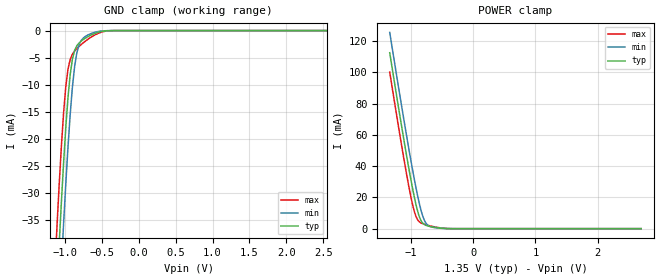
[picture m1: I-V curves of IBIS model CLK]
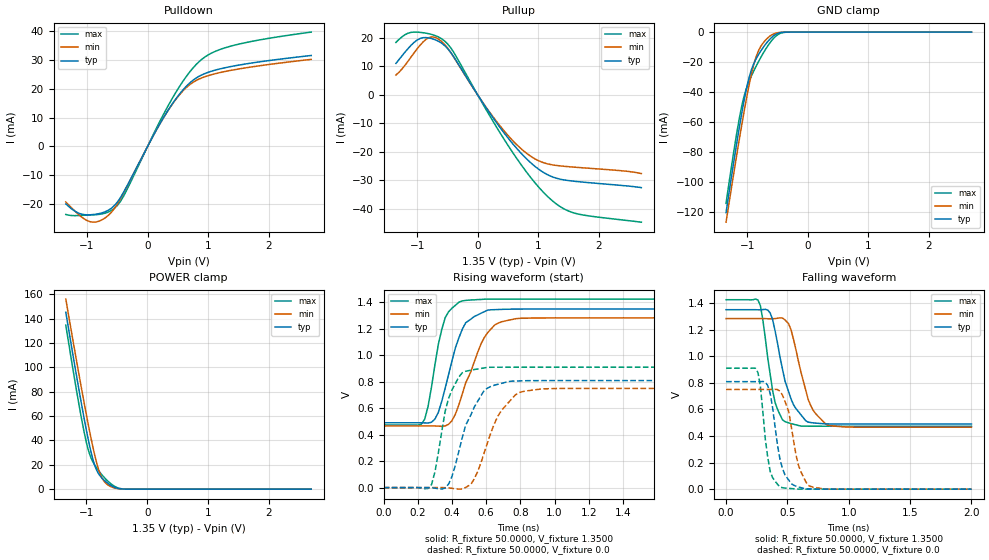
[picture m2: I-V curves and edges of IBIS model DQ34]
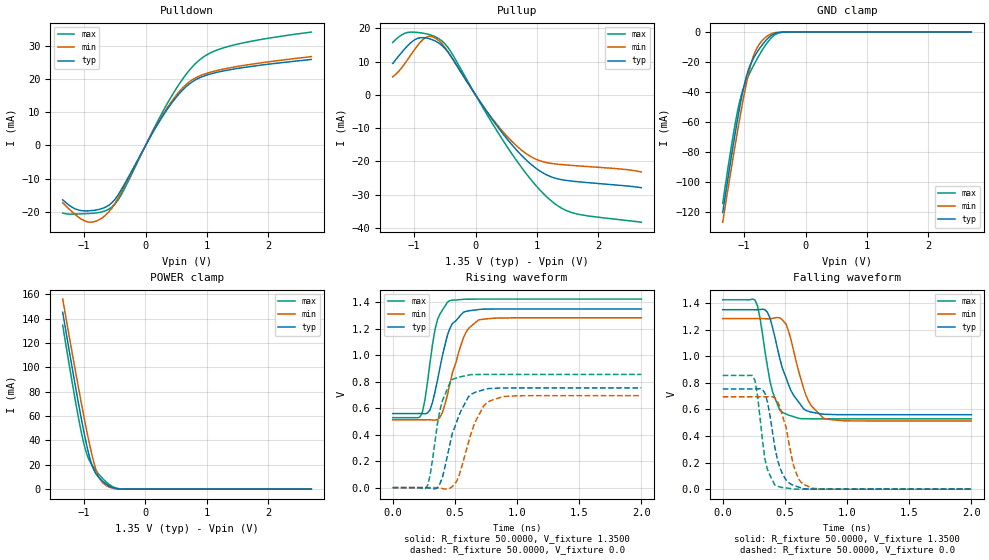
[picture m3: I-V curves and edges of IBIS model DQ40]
|   IBIS file usslh2g16ec.ibs
[IBIS ver] 3.2
[File name] usslh2g16ec.ibs
[File Rev] 1.06
[Date] Dec. 08th, 2020
[Source] File generated by UniIC.
[Notes]  Rev 1.0: 03/21/2019
   - New model generated.
   Rev 1.01: 06/12/2019
   - Adjust DQ34/DQ40 model rising waveform and
   falling waveform.
   Rev 1.02: 10/03/2019
   - 1. Modify CLK and INPUT model GND Clamp and POWER Clamp.
   - 2. Moidfy DQ34 and DQ40 model.
   Rev 1.03: 12/06/2019
   - Modified all ODT model content. Change to use v1.0 value.
   Rev 1.04: 12/06/2019
   - Update RLC information.
   Rev 1.05: 12/23/2019
   - Modified content of all ODT models.
   Rev 1.06: 12/08/2020
   - update 95c data.
[Disclaimer]  THESE IBIS MODELS ARE PROVIDED "AS IS" WITH NO WARRANTY
   AND UniIC IS NOT RESPONSIBLE FOR ANY PROBLEMS THIS MODEL
   MAY CAUSE TO THE CUSTOMERS. THESE MODELS ARE SUBJECT TO CHANGE
   WITHOUT ANY NOTICE.
[Copyright] Copyright 2020. UniIC All rights reserved.
|   Component: SCB13H2G160EF
|   2G DDR3L SDRAM X16
|   VDD/VDDQ : 1.35V
[Component] SCB13H2G160EF
[Manufacturer]  UniIC.
[Package]
|   typ   min   max
R_pkg   0.624   0.464   0.798
L_pkg   1.862nH   1.145nH   3.060nH
C_pkg   0.529pF   0.376pF   0.813pF
[Pin]   signal_name   model_name   R_pin   L_pin   C_pin
A1   VDDQ   POWER
A2   DQU5   DQ   0.782   2.212nH   0.593pF
A3   DQU7   DQ   0.720   1.890nH   0.554pF
A7   DQU4   DQ   0.536   1.899nH   0.568pF
A8   VDDQ   POWER
A9   VSS   GND
B1   VSS   GND
B2   VDD   POWER
B3   VSS   GND
B7   DQSUB   DQ   0.674   1.734nH   0.587pF
B8   DQU6   DQ   0.791   2.263nH   0.576pF
B9   VSS   GND
C1   VDDQ   POWER
C2   DQU3   DQ   0.669   1.891nH   0.538pF
C3   DQU1   DQ   0.577   1.375nH   0.563pF
C7   DQSU   DQ   0.678   1.680nH   0.578pF
C8   DQU2   DQ   0.759   2.136nH   0.557pF
C9   VDDQ   POWER
D1   VSS   GND
D2   VDDQ   POWER
D3   DMU   DQ   0.570   1.24nH   0.562pF
D7   DQU0   DQ   0.511   1.214nH   0.532pF
D8   VSS   GND
D9   VDD   POWER
E1   VSS   GND
E2   VSS   GND
E3   DQL0   DQ   0.527   1.246nH   0.558pF
E7   DML   DQ   0.528   1.181nH   0.559pF
E8   VSS   GND
E9   VDDQ   POWER
F1   VDDQ   POWER
F2   DQL2   DQ   0.649   1.448nH   0.569pF
F3   DQSL   DQ   0.600   1.602nH   0.552pF
F7   DQL1   DQ   0.503   1.145nH   0.544pF
F8   DQL3   DQ   0.610   1.407nH   0.554pF
F9   VSS   GND
G1   VSS   GND
G2   DQL6   DQ   0.589   1.311nH   0.543pF
G3   DQSLB   DQ   0.595   1.638nH   0.544pF
G7   VDD   POWER
G8   VSS   GND
G9   VSS   GND
H1   VREFQ   POWER
H2   VDD   POWER
H3   DQL4   DQ   0.550   1.26nH   0.565pF
H7   DQL7   DQ   0.587   1.352nH   0.567pF
H8   DQL5   DQ   0.731   1.671nH   0.576pF
H9   VDDQ   POWER
J2   VSS   GND
J3   RASB   INPUT   0.464   1.391nH   0.444pF
J7   CK   CLK   0.472   1.167nH   0.376pF
J8   VSS   GND
K1   ODT   INPUT   0.628   2.345nH   0.451pF
K2   VDD   POWER
K3   CASB   INPUT   0.476   1.52nH   0.452pF
K7   CKB   CLK   0.467   1.314nH   0.389pF
K8   VDD   POWER
K9   CKE   INPUT   0.685   2.271nH   0.502pF
L2   CSB   INPUT   0.576   2.026nH   0.444pF
L3   WEB   INPUT   0.495   1.669nH   0.437pF
L7   A10   INPUT   0.491   1.335nH   0.448pF
L8   ZQ   INPUT   0.652   1.676nH   0.497pF
M1   VSS   GND
M2   BA0   INPUT   0.601   2.209nH   0.446pF
M3   BA2   INPUT   0.565   1.827nH   0.450pF
M9   VSS   GND
N1   VDD   POWER
N2   A3   INPUT   0.669   2.297nH   0.501pF
N3   A0   INPUT   0.546   1.663nH   0.460pF
N7   A12   INPUT   0.545   1.919nH   0.480pF
N8   BA1   INPUT   0.671   2.186nH   0.501pF
N9   VDD   POWER
P1   VSS   GND
P2   A5   INPUT   0.701   2.412nH   0.530pF
P3   A2   INPUT   0.614   2.102nH   0.542pF
P7   A1   INPUT   0.582   2.095nH   0.521pF
P8   A4   INPUT   0.686   2.439nH   0.542pF
P9   VSS   GND
R1   VSS   GND
R2   A7   INPUT   0.763   2.744nH   0.587pF
R3   A9   INPUT   0.673   2.375nH   0.534pF
R7   A11   INPUT   0.633   2.347nH   0.507pF
R8   A6   INPUT   0.761   2.758nH   0.599pF
R9   VDD   POWER
T1   VSS   GND
T2   RESETB   INPUT   0.798   2.031nH   0.813pF
T3   A13   INPUT   0.752   2.571nH   0.549pF
T7   A14   INPUT   0.717   2.562nH   0.523pF
T8   A8   INPUT   0.798   3.060nH   0.580pF
T9   VSS   GND
|**********************DIFF PIN*********************************************
[Diff_pin]   inv_pin   vdiff   tdelay_typ   tdelay_min   tdelay_max
   J7   K7   0V   0ns   NA   NA
   F3   G3   0V   0ns   NA   NA
   C7   B7   0V   0ns   NA   NA
|   Model Selector
[Model Selector]  DQ
DQ34   34ohm data I/O without ODT
DQ40   40ohm data I/O without ODT
ODT20   Data input with 20ohm ODT
ODT30   Data input with 30ohm ODT
ODT40   Data input with 40ohm ODT
ODT60   Data input with 60ohm ODT
ODT120   Data input with 120ohm ODT
| Models and submodels in the file (14): CLK (Input), INPUT (Input), DQ34 (I/O), DQ40 (I/O), ODT20 (Input), ODT30 (Input), ODT40 (Input), ODT60 (Input), ODT120 (Input), 20ohm_ODT (Dynamic_clamp), 30ohm_ODT (Dynamic_clamp), 40ohm_ODT (Dynamic_clamp), 60ohm_ODT (Dynamic_clamp), 120ohm_ODT (Dynamic_clamp)
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|   Model CLK
[Model]  CLK
Model_type   Input
Polarity   Non-Inverting
Vinl =   0.5750V
Vinh =   0.7750V
| variable   typ   min   max
C_comp   0.4980pF   0.4480pF   0.5480pF
| variable   typ   min   max
[Temperature Range]   45.000   95.000   0.000
| variable   typ   min   max
[Voltage Range]   1.35V   1.283V   1.4250V
| variable   typ   min   max
[POWER Clamp Reference] 1.35V   1.283V   1.4250V
| variable   typ   min   max
[GND Clamp Reference]   0.000V   0.000V   0.000V
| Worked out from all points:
|   GND clamp passes 1 mA (typ) near -0.67 V on its own axis
|   POWER clamp passes 1 mA (typ) near -0.64 V on its own axis
[GND_clamp]
|Voltage   I(typ)   I(min)   I(max)
-1.35V    -119.8mA   -132.6mA   -107.8mA
-1.11V    -47.85mA   -60.25mA   -36.41mA
-1.08V    -39.66mA   -51.82mA   -28.64mA
-1.05V    -31.85mA   -43.65mA   -21.5mA
-1.02V    -24.55mA   -35.8mA    -15.28mA
-990mV    -17.97mA   -28.39mA   -10.4mA
-930mV    -8.108mA   -15.48mA   -5.33mA
-870mV    -3.674mA   -6.627mA   -3.777mA
-810mV    -2.286mA   -2.636mA   -2.929mA
-720mV    -1.363mA   -1.035mA   -1.906mA
-390mV    -14.42uA   -7.911uA   -27.31uA
2.7V      0A         0A         0A
[POWER_clamp]
|Voltage   I(typ)   I(min)   I(max)
-1.34V    112.5mA    125.5mA    100.1mA
-1.2V     77.82mA    90.79mA    65.48mA
-1.1V     53.88mA    66.67mA    41.81mA
-1.02V    35.69mA    48.08mA    24.36mA
-960mV    23.14mA    34.83mA    13.32mA
-900mV    12.44mA    22.6mA     6.231mA
-840mV    5.342mA    12.19mA    3.716mA
-780mV    2.549mA    5.064mA    2.758mA
-720mV    1.647mA    1.95mA     2.065mA
-600mV    737.4uA    566.8uA    984.4uA
-360mV    19.27uA    12.95uA    28.6uA
2.7V      0A         0A         0A
|   Model DQ34
[Model]  DQ34
Model_type I/O
Polarity   Non-Inverting
Enable   Active-High
Vinl =   0.5750V
Vinh =   0.7750V
Vmeas =  0.6750V
Cref =   0.0F
Rref =   25.0000
Vref =   0.6750V
| variable   typ   min   max
C_comp   1.0500pF   1.0000pF   1.1000pF
| variable   typ   min   max
[Temperature Range]   45.000   95.000   0.000
| variable   typ   min   max
[Voltage Range]   1.35V   1.283V   1.4250V
| variable   typ   min   max
[Pullup Reference]   1.35V   1.283V   1.4250V
| variable   typ   min   max
[Pulldown Reference]   0.000V   0.000V   0.000V
| variable   typ   min   max
[POWER Clamp Reference] 1.35V   1.283V   1.4250V
| variable   typ   min   max
[GND Clamp Reference]   0.000V   0.000V   0.000V
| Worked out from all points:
|   slope of the pulldown table from 0 to 0.203 V, typ, clamps not added: 25.8 ohm
|   slope of the pullup table from 0 to 0.203 V, typ, clamps not added: 31.3 ohm
|   GND clamp passes 1 mA (typ) near -0.50 V on its own axis
|   POWER clamp passes 1 mA (typ) near -0.51 V on its own axis
|   rising waveform, R_fixture 50.0000, V_fixture 1.3500: 20-80 % time 112ps typ, 142ps min, 82.2ps max; typ from 0.49 V to 1.35 V
|   rising waveform, R_fixture 50.0000, V_fixture 0.0: 20-80 % time 130ps typ, 142ps min, 87.7ps max; typ from 0 V to 0.809 V
|   falling waveform, R_fixture 50.0000, V_fixture 1.3500: 20-80 % time 135ps typ, 138ps min, 91.5ps max; typ from 1.35 V to 0.49 V
|   falling waveform, R_fixture 50.0000, V_fixture 0.0: 20-80 % time 84.9ps typ, 97.5ps min, 66ps max; typ from 0.809 V to 0 V
[Pulldown]
|Voltage   I(typ)   I(min)   I(max)
-1.35V    -19.97mA   -19.29mA   -23.65mA
-1.15V    -23.09mA   -23.47mA   -24.03mA
-950mV    -23.77mA   -26.17mA   -23.85mA
-650mV    -22.21mA   -24.01mA   -22.83mA
-500mV    -19.4mA    -20.05mA   -20.54mA
-400mV    -16.07mA   -16.29mA   -17.41mA
100mV     3.983mA    3.979mA    4.397mA
400mV     14.55mA    14.43mA    16.42mA
650mV     21.14mA    20.67mA    24.63mA
900mV     24.9mA     23.86mA    30.36mA
1.45V     28.05mA    26.72mA    35.27mA
2.7V      31.59mA    30.25mA    39.73mA
[Pullup]
|Voltage   I(typ)   I(min)   I(max)
-1.35V    11.07mA    6.98mA     18.44mA
-1.15V    16.28mA    11.86mA    21.68mA
-1V       19.27mA    16.18mA    22.06mA
-850mV    20.14mA    19.59mA    21.68mA
-700mV    19.35mA    20.18mA    20.83mA
-400mV    13.51mA    13.42mA    15.11mA
150mV     -4.843mA   -4.665mA   -5.558mA
550mV     -16.41mA   -15.39mA   -19.33mA
900mV     -24.27mA   -21.87mA   -29.66mA
1.2V      -28.46mA   -24.4mA    -36.56mA
1.6V      -30.3mA    -25.34mA   -41.48mA
2.7V      -32.52mA   -27.58mA   -44.65mA
[GND_clamp]
|Voltage   I(typ)   I(min)   I(max)
-1.35V    -120.2mA   -126.6mA   -114.1mA
-1.23V    -88.34mA   -95.9mA    -81.52mA
-1.14V    -65.66mA   -73.61mA   -59.5mA
-1.05V    -45.07mA   -52.44mA   -42.33mA
-990mV    -33.57mA   -39.39mA   -34.75mA
-930mV    -24.92mA   -27.79mA   -29.03mA
-840mV    -16.77mA   -14.89mA   -21.65mA
-750mV    -10.97mA   -7.891mA   -14.99mA
-630mV    -4.83mA    -2.8mA     -7.385mA
-510mV    -1.116mA   -502.7uA   -2.115mA
-360mV    -46.72uA   -22.21uA   -95.74uA
2.7V      0A         0A         0A
[POWER_clamp]
|Voltage   I(typ)   I(min)   I(max)
-1.34V    145.4mA    156.2mA    134.8mA
-1.12V    80.7mA     93.36mA    68.62mA
-1.04V    58.61mA    71.47mA    47.35mA
-980mV    43.17mA    55.66mA    34.17mA
-940mV    33.8mA     45.58mA    27.64mA
-880mV    22.09mA    31.49mA    21.14mA
-800mV    12.67mA    16.11mA    15.22mA
-740mV    8.89mA     8.743mA    11.48mA
-660mV    5.266mA    3.989mA    7.183mA
-520mV    1.208mA    721.2uA    1.904mA
-360mV    46.31uA    30.1uA     72.07uA
2.7V      0A         0A         0A
[Ramp]
| variable   typ   min   max
dV/dt_r  0.4853/0.1200n   0.4499/0.1421n   0.5459/88.0013p
dV/dt_f  0.5160/0.1249n   0.4903/0.1383n   0.5710/91.2670p
R_load = 50.0000
[Rising Waveform]
R_fixture= 50.0000
V_fixture= 1.3500
V_fixture_min= 1.2830
V_fixture_max= 1.4250
L_fixture= 0.0H
C_fixture= 0.0F
|time   V(typ)   V(min)   V(max)
0s        490mV      465.8mV    473.3mV
240ps     489.3mV    465.8mV    516.5mV
260ps     488.1mV    465.8mV    613.9mV
300ps     517.4mV    465.9mV    927.6mV
360ps     751.1mV    466.1mV    1.284V
400ps     958.8mV    505.9mV    1.356V
460ps     1.196V     706.9mV    1.411V
590ps     1.33V      1.136V     1.424V
690ps     1.347V     1.253V     1.425V
2ns       1.35V      1.283V     1.425V
[Rising Waveform]
R_fixture= 50.0000
V_fixture= 0.0
V_fixture_min= 0.0
V_fixture_max= 0.0
L_fixture= 0.0H
C_fixture= 0.0F
|time   V(typ)   V(min)   V(max)
0s        0V         0V         0V
280ps     -938.2uV   -50.3uV    22.28mV
380ps     26.61mV    -2.235mV   674.6mV
440ps     273.8mV    -11.77mV   836mV
480ps     471.5mV    1.462mV    879.3mV
530ps     607.6mV    65.88mV    892.1mV
590ps     737mV      269.6mV    905mV
670ps     781.4mV    542.8mV    909.7mV
790ps     806.3mV    717.3mV    909.9mV
2ns       808.8mV    749.8mV    909.9mV
[Falling Waveform]
R_fixture= 50.0000
V_fixture= 1.3500
V_fixture_min= 1.2830
V_fixture_max= 1.4250
L_fixture= 0.0H
C_fixture= 0.0F
|time   V(typ)   V(min)   V(max)
0s        1.35V      1.283V     1.425V
260ps     1.349V     1.283V     1.423V
300ps     1.351V     1.283V     1.272V
360ps     1.325V     1.282V     862.1mV
400ps     1.189V     1.283V     650.3mV
480ps     815.1mV    1.274V     508.2mV
530ps     677.3mV    1.198V     492.8mV
670ps     503.9mV    672.9mV    473.6mV
830ps     490.9mV    481mV      473.3mV
2ns       490mV      465.8mV    473.3mV
[Falling Waveform]
R_fixture= 50.0000
V_fixture= 0.0
V_fixture_min= 0.0
V_fixture_max= 0.0
L_fixture= 0.0H
C_fixture= 0.0F
|time   V(typ)   V(min)   V(max)
0s        808.8mV    749.8mV    909.9mV
260ps     808.5mV    749.8mV    876.9mV
280ps     808.7mV    749.9mV    772.8mV
320ps     805.7mV    749.8mV    376.4mV
360ps     718.4mV    749.6mV    132.1mV
440ps     222mV      736.8mV    15.22mV
510ps     69.56mV    586.8mV    5.903mV
590ps     16.7mV     179.9mV    358.3uV
670ps     1.797mV    27.86mV    -70.56uV
2ns       1.662uV    -1.338uV   1.858uV
|   Model DQ40
[Model]  DQ40
Model_type I/O
Polarity   Non-Inverting
Enable   Active-High
Vinl =   0.5750V
Vinh =   0.7750V
Vmeas =  0.6750V
Cref =   0.0F
Rref =   25.0000
Vref =   0.6750V
| variable   typ   min   max
C_comp   1.0500pF   1.0000pF   1.1000pF
| variable   typ   min   max
[Temperature Range]   45.000   95.000   0.000
| variable   typ   min   max
[Voltage Range]   1.35V   1.283V   1.4250V
| variable   typ   min   max
[Pullup Reference]   1.35V   1.283V   1.4250V
| variable   typ   min   max
[Pulldown Reference]   0.000V   0.000V   0.000V
| variable   typ   min   max
[POWER Clamp Reference] 1.35V   1.283V   1.4250V
| variable   typ   min   max
[GND Clamp Reference]   0.000V   0.000V   0.000V
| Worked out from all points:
|   slope of the pulldown table from 0 to 0.203 V, typ, clamps not added: 31 ohm
|   slope of the pullup table from 0 to 0.203 V, typ, clamps not added: 36.5 ohm
|   GND clamp passes 1 mA (typ) near -0.50 V on its own axis
|   POWER clamp passes 1 mA (typ) near -0.51 V on its own axis
|   rising waveform, R_fixture 50.0000, V_fixture 1.3500: 20-80 % time 117ps typ, 137ps min, 87.4ps max; typ from 0.56 V to 1.35 V
|   rising waveform, R_fixture 50.0000, V_fixture 0.0: 20-80 % time 143ps typ, 148ps min, 98.7ps max; typ from 0 V to 0.754 V
|   falling waveform, R_fixture 50.0000, V_fixture 1.3500: 20-80 % time 156ps typ, 141ps min, 104ps max; typ from 1.35 V to 0.56 V
|   falling waveform, R_fixture 50.0000, V_fixture 0.0: 20-80 % time 94.4ps typ, 106ps min, 71.5ps max; typ from 0.754 V to 0 V
[Pulldown]
|Voltage   I(typ)   I(min)   I(max)
-1.35V    -16.31mA   -17.17mA   -20.27mA
-1.15V    -19.01mA   -20.69mA   -20.6mA
-950mV    -19.64mA   -22.91mA   -20.44mA
-650mV    -18.49mA   -20.9mA    -19.57mA
-500mV    -16.2mA    -17.43mA   -17.61mA
-400mV    -13.43mA   -14.16mA   -14.92mA
100mV     3.324mA    3.459mA    3.769mA
400mV     12.09mA    12.6mA     14.08mA
650mV     17.49mA    18.14mA    21.11mA
900mV     20.49mA    21.04mA    26.02mA
1.45V     22.99mA    23.58mA    30.23mA
2.7V      25.82mA    26.68mA    34.05mA
[Pullup]
|Voltage   I(typ)   I(min)   I(max)
-1.35V    9.49mA     5.47mA     15.8mA
-1.15V    13.95mA    9.5mA      18.59mA
-1V       16.52mA    13.51mA    18.91mA
-850mV    17.26mA    16.81mA    18.58mA
-700mV    16.59mA    17.5mA     17.86mA
-400mV    11.58mA    11.64mA    12.95mA
150mV     -4.151mA   -4.025mA   -4.764mA
550mV     -14.06mA   -13.18mA   -16.57mA
900mV     -20.81mA   -18.54mA   -25.42mA
1.2V      -24.4mA    -20.49mA   -31.34mA
1.65V     -26.07mA   -21.3mA    -35.79mA
2.7V      -27.88mA   -23.18mA   -38.27mA
[GND_clamp]
|Voltage   I(typ)   I(min)   I(max)
-1.35V    -120.2mA   -126.6mA   -114.1mA
-1.23V    -88.34mA   -95.9mA    -81.52mA
-1.14V    -65.66mA   -73.61mA   -59.5mA
-1.05V    -45.07mA   -52.44mA   -42.33mA
-990mV    -33.57mA   -39.39mA   -34.75mA
-930mV    -24.92mA   -27.79mA   -29.03mA
-840mV    -16.77mA   -14.89mA   -21.65mA
-750mV    -10.97mA   -7.891mA   -14.99mA
-630mV    -4.83mA    -2.8mA     -7.385mA
-510mV    -1.116mA   -502.7uA   -2.115mA
-360mV    -46.72uA   -22.21uA   -95.74uA
2.7V      0A         0A         0A
[POWER_clamp]
|Voltage   I(typ)   I(min)   I(max)
-1.34V    145.4mA    156.2mA    134.8mA
-1.12V    80.7mA     93.36mA    68.62mA
-1.04V    58.61mA    71.47mA    47.35mA
-980mV    43.17mA    55.66mA    34.17mA
-940mV    33.8mA     45.58mA    27.64mA
-880mV    22.09mA    31.49mA    21.14mA
-800mV    12.67mA    16.11mA    15.22mA
-740mV    8.89mA     8.743mA    11.48mA
-660mV    5.266mA    3.989mA    7.183mA
-520mV    1.208mA    721.2uA    1.904mA
-360mV    46.31uA    30.1uA     72.07uA
2.7V      0A         0A         0A
[Ramp]
| variable   typ   min   max
dV/dt_r  0.4523/0.1331n   0.4170/0.1476n   0.5132/98.6582p
dV/dt_f  0.4740/0.1462n   0.4620/0.1406n   0.5376/0.1040n
R_load = 50.0000
[Rising Waveform]
R_fixture= 50.0000
V_fixture= 1.3500
V_fixture_min= 1.2830
V_fixture_max= 1.4250
L_fixture= 0.0H
C_fixture= 0.0F
|time   V(typ)   V(min)   V(max)
0s        560mV      513mV      529mV
220ps     560.2mV    513mV      535mV
260ps     557.7mV    513mV      666.2mV
300ps     588.3mV    513mV      945.1mV
360ps     811.2mV    513.9mV    1.269V
400ps     998.2mV    568.3mV    1.342V
460ps     1.203V     782.9mV    1.414V
570ps     1.326V     1.135V     1.423V
690ps     1.346V     1.267V     1.425V
2ns       1.35V      1.283V     1.425V
[Rising Waveform]
R_fixture= 50.0000
V_fixture= 0.0
V_fixture_min= 0.0
V_fixture_max= 0.0
L_fixture= 0.0H
C_fixture= 0.0F
|time   V(typ)   V(min)   V(max)
0s        0V         0V         0V
280ps     -1.179mV   -56.53uV   13.96mV
300ps     -4.246mV   187.6uV    90.12mV
380ps     29.65mV    -3.414mV   585.2mV
480ps     412mV      8.256mV    818.1mV
530ps     539mV      81.09mV    834.6mV
610ps     688.6mV    344.4mV    850.3mV
730ps     739.3mV    614.3mV    855.3mV
790ps     749.5mV    657.8mV    855.3mV
2ns       753.8mV    695mV      855.3mV
[Falling Waveform]
R_fixture= 50.0000
V_fixture= 1.3500
V_fixture_min= 1.2830
V_fixture_max= 1.4250
L_fixture= 0.0H
C_fixture= 0.0F
|time   V(typ)   V(min)   V(max)
0s        1.35V      1.283V     1.425V
260ps     1.349V     1.283V     1.423V
300ps     1.351V     1.283V     1.288V
360ps     1.33V      1.282V     921.4mV
400ps     1.219V     1.284V     736.9mV
480ps     909.4mV    1.273V     577.7mV
530ps     784.3mV    1.187V     556.8mV
670ps     592mV      705mV      529.8mV
810ps     563.8mV    534.8mV    529mV
2ns       560mV      513mV      529mV
[Falling Waveform]
R_fixture= 50.0000
V_fixture= 0.0
V_fixture_min= 0.0
V_fixture_max= 0.0
L_fixture= 0.0H
C_fixture= 0.0F
|time   V(typ)   V(min)   V(max)
0s        753.8mV    695mV      855.3mV
260ps     753.4mV    695mV      816mV
340ps     720.5mV    694.7mV    224.2mV
380ps     555.1mV    696.2mV    104.6mV
420ps     311.7mV    686.9mV    30.29mV
460ps     162.1mV    620.7mV    15.94mV
510ps     68.5mV     464.9mV    9.258mV
570ps     27.95mV    178.1mV    1.041mV
650ps     3.55mV     36.84mV    -38.75uV
2ns       5.419uV    1.261uV    1.263uV
